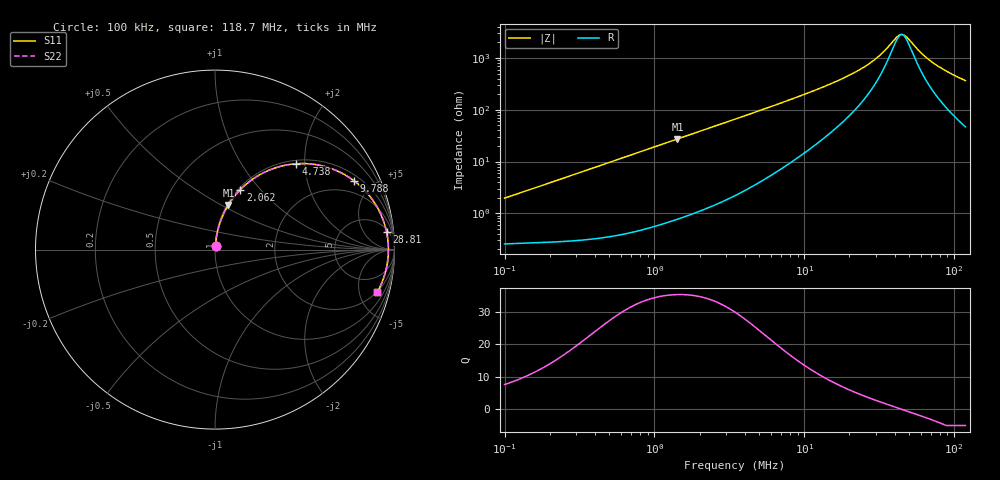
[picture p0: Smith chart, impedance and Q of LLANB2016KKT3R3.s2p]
! LLANB2016KKT3R3  S-PARAMETER MODEL  ( General Type )
! Model Generated by TAIYO YUDEN Corporation (http://www.ty-top.com)
! Version 1.0
! TAIYO YUDEN Control No. 120417NG38SB-FKC
! Copyright(c) 2012 TAIYO YUDEN CO.,LTD. All Rights Reserved.
! Product Description (link to TY-COMPAS)
! https://ds.yuden.co.jp/TYCOMPAS/or/detail?pn=LLANB2016KKT3R3M&u=M
! Products Name : Inductors
! Characteristics :
!  Inductance : 3.3 uH , SRF(min) : -Hz , DC Resistance(max) : 0.255 Ohm
!  Rated Current : Saturation :1150 mA , Temp Rise : 1200 mA (40 degC)
!  Case Size : 2.0 x 1.6 / 0.079 x 0.063 [mm/inch] , Thickness : 1 / 0.039 [mm/inch]
!  (Conditions: Temperature = 25 degC , DC Bias Current/Voltage = 0A / 0V)
! External Node Assignments :
!  1  o---GGG---o  2
! GND o---------o GND
! Frequency Range : 0.1MHz  -  118.695536MHz  [ 402 STEP ]
# MHz S RI R 50
! Freq[MHz].  S11 Real  S11 Imag  S21 Real  S21 Imag  S12 Real  S12 Imag  S22 Real  S22 Imag
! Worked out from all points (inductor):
!   401 points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, 100 kHz to 118.7 MHz, reference 50 ohm
!   read as one part in series: L = 3.09 uH near 103.6 kHz
!   highest Q = 35.4 at 1.422 MHz (marker M1), where L = 3.04 uH
!   self-resonance near 44.65 MHz
!   S11 on the Smith chart (normalised r, x): 100 kHz: 1.01, +0.04; 2.062 MHz: 1.02, +0.79; 4.738 MHz: 1.07, +1.81; 9.788 MHz: 1.28, +3.87; 28.81 MHz: 7, +17; 118.7 MHz: 1.94, -7.27
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0.1  0.00293 0.0194  0.9971 -0.0194  0.9971 -0.0194  0.00293 0.0194
0.327316  0.00694 0.0624  0.9931 -0.0624  0.9931 -0.0624  0.00694 0.0624
0.618966  0.0177 0.1163  0.9823 -0.1163  0.9823 -0.1163  0.0177 0.1163
1.07136  0.0455 0.1945  0.9545 -0.1945  0.9545 -0.1945  0.0455 0.1945
1.422044  0.0748 0.2493  0.9252 -0.2493  0.9252 -0.2493  0.0748 0.2493
2.062152  0.1408 0.3337  0.8592 -0.3337  0.8592 -0.3337  0.1408 0.3337
3.445222  0.3073 0.445  0.6927 -0.445  0.6927 -0.445  0.3073 0.445
4.737691  0.4532 0.4784  0.5468 -0.4784  0.5468 -0.4784  0.4532 0.4784
6.631356  0.616 0.4616  0.384 -0.4616  0.384 -0.4616  0.616 0.4616
9.788052  0.7741 0.3836  0.2259 -0.3836  0.2259 -0.3836  0.7741 0.3836
11.27678  0.8181 0.3463  0.1819 -0.3463  0.1819 -0.3463  0.8181 0.3463
19.51882  0.9243 0.1956  0.0757 -0.1956  0.0757 -0.1956  0.9243 0.1956
24.13719  0.9447 0.1415  0.0553 -0.1415  0.0553 -0.1415  0.9447 0.1415
28.81028  0.9558 0.0989  0.0442 -0.0989  0.0442 -0.0989  0.9558 0.0989
36.91074  0.9642 0.0422  0.0358 -0.0422  0.0358 -0.0422  0.9642 0.0422
42.52471  0.966 0.0108  0.034 -0.0108  0.034 -0.0108  0.966 0.0108
44.84352  0.9662 -0.000982  0.0338 0.000982  0.0338 0.000982  0.9662 -0.000982
46.45921  0.9661 -0.00881  0.0339 0.00881  0.0339 0.00881  0.9661 -0.00881
60.58472  0.9614 -0.0683  0.0386 0.0683  0.0386 0.0683  0.9614 -0.0683
71.04572  0.9547 -0.1053  0.0453 0.1053  0.0453 0.1053  0.9547 -0.1053
91.02131  0.9368 -0.1661  0.0632 0.1661  0.0632 0.1661  0.9368 -0.1661
118.6955  0.9045 -0.2365  0.0955 0.2365  0.0955 0.2365  0.9045 -0.2365
